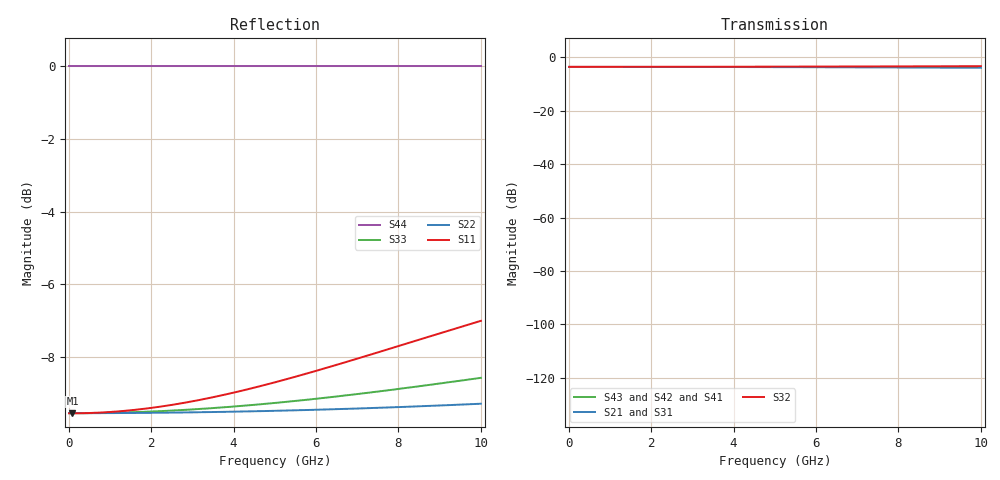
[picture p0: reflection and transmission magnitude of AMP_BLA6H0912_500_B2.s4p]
! Created Tue Apr 27 00:36:48 2010
# ghz S ma R 50
! 4 Port Network Data from SP1.SP block
! freq  magS11  angS11  magS12  angS12  magS13  angS13  magS14  angS14
!  magS21  angS21  magS22  angS22  magS23  angS23  magS24  angS24
!  magS31  angS31  magS32  angS32  magS33  angS33  magS34  angS34
!  magS41  angS41  magS42  angS42  magS43  angS43  magS44  angS44
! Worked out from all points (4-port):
!   1000 points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, 10 MHz to 10 GHz, reference 50 ohm
!   strongest paths, dB at 10 MHz, 2.51 GHz, 5.01 GHz, 7.51 GHz, 10 GHz:
!     S32: -3.5, -3.5, -3.4, -3.4, -3.3
!     S21: -3.5, -3.5, -3.6, -3.7, -3.9
!     S31: -3.5, -3.6, -3.7, -3.9, -4.1
!     S43: -, -, -, -, -
!     S42: -, -, -, -, -
!     S41: -, -, -, -, -
!   lowest |S11| = -9.5 dB at 90 MHz (marker M1), VSWR 2.00, Z = 25 + j0.231 ohm
!   |S11| at or under -10 dB: nowhere
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0.01  0.3331 179.9  0.6666 -0.0  0.6666 -0.0  3.093e-12 -172.0
      0.6666 -0.0  0.3333 180.0  0.6667 0.0  3.093e-12 -172.1
      0.6666 -0.0  0.6667 0.0  0.3333 179.9  3.094e-12 -172.1
      3.093e-12 -172.0  3.094e-12 -172.1  3.094e-12 -172.1  1 0.0
0.09  0.3331 179.3  0.6666 -0.1  0.6665 -0.2  5.521e-13 -82.7
      0.6666 -0.1  0.3333 179.8  0.6667 0.0  5.523e-13 -83.3
      0.6665 -0.2  0.6667 0.0  0.3333 179.5  5.523e-13 -83.4
      5.521e-13 -82.8  5.523e-13 -83.3  5.523e-13 -83.3  1 0.0
2.26  0.3405 162.5  0.665 -2.9  0.6641 -6.0  1.379e-14 -82.9
      0.665 -2.9  0.3337 174.3  0.6679 0.0  1.364e-14 -100.8
      0.6641 -6.0  0.6679 0.0  0.3355 168.1  1.372e-14 -104.4
      1.374e-14 -83.2  1.36e-14 -99.5  1.348e-14 -99.4  1 0.0
4.72  0.3639 144.8  0.6603 -5.9  0.6562 -12.4  3.119e-15 129.6
      0.6603 -5.9  0.3355 168.2  0.6717 -0.0  1.989e-15 98.2
      0.6562 -12.4  0.6717 -0.0  0.3431 155.6  1.979e-15 81.7
      3.324e-15 133.2  1.973e-15 87.9  2.037e-15 69.6  1 -0.0
6.07  0.382 136.1  0.6563 -7.6  0.6498 -15.9  1.452e-14 115.5
      0.6563 -7.6  0.337 164.9  0.6748 -0.1  1.194e-14 76.2
      0.6498 -15.9  0.6748 -0.1  0.3492 149.1  1.204e-14 67.8
      1.437e-14 113.8  1.188e-14 76.9  1.214e-14 66.9  1 -0.0
7.49  0.4038 127.8  0.6513 -9.3  0.6415 -19.5  8.205e-15 128.6
      0.6513 -9.3  0.3389 161.5  0.6786 -0.2  4.574e-15 86.4
      0.6415 -19.5  0.6786 -0.2  0.3568 142.6  4.29e-15 70.7
      8.097e-15 126.5  4.542e-15 84.2  4.587e-15 61.3  1 -0.0
10  0.4465 115.0  0.6406 -12.1  0.6238 -25.7  1.137e-15 1.8
    0.6406 -12.1  0.3434 155.7  0.6865 -0.6  1.421e-15 -0.9
    0.6238 -25.7  0.6865 -0.6  0.3727 131.8  1.425e-15 4.1
    1.079e-15 13.8  1.812e-15 -1.3  2.238e-15 -0.7  1 -0.0
